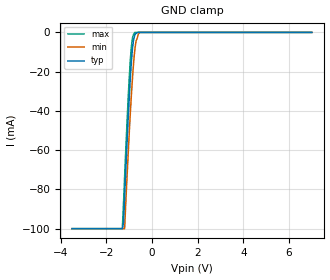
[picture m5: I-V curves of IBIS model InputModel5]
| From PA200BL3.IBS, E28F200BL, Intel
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|*********************Input Model 5*********************************
[Model]   InputModel5
Model_type   Input
|   Model for WE# pin.
Vinl = 0.8V
Vinh = 2.0V
|Variable   Typ   Min   Max
C_comp   5.61p   NA   7.6p
[Voltage Range]   3.3V   3.0V   3.6V
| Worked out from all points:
|   GND clamp passes 1 mA (typ) near -0.74 V on its own axis
[GND_clamp]
|Voltage  I(typ)   I(min)   I(max)
-3.5V     -100mA     -100mA     -100mA
-1.3V     -100mA     -100mA     -100mA
-1.25V    -97.24mA   -100mA     -87.43mA
-1.2V     -83.72mA   -100mA     -73.55mA
-1.05V    -45.35mA   -63.18mA   -34.89mA
-950mV    -23.26mA   -41.1mA    -13.99mA
-900mV    -14.29mA   -31.06mA   -6.696mA
-850mV    -7.575mA   -22.27mA   -2.52mA
-750mV    -1.185mA   -8.518mA   0A
-700mV    -435.9uA   -4.41mA    0A
-550mV    0A         0A         0A
7V        0A         0A         0A
[Power_clamp]
| Input buffer circuits of this product do not intrinsically
| require a [Power_clamp] definition.  This zero current
| [Power_clamp] table is provided for the compatibility with
| some IBIS parsers.
|Voltage  I(typ)   I(min)   I(max)
-3.3V     0A         0A         0A
0V        0A         0A         0A
3.3V      0A         0A         0A
7V        0A         0A         0A
